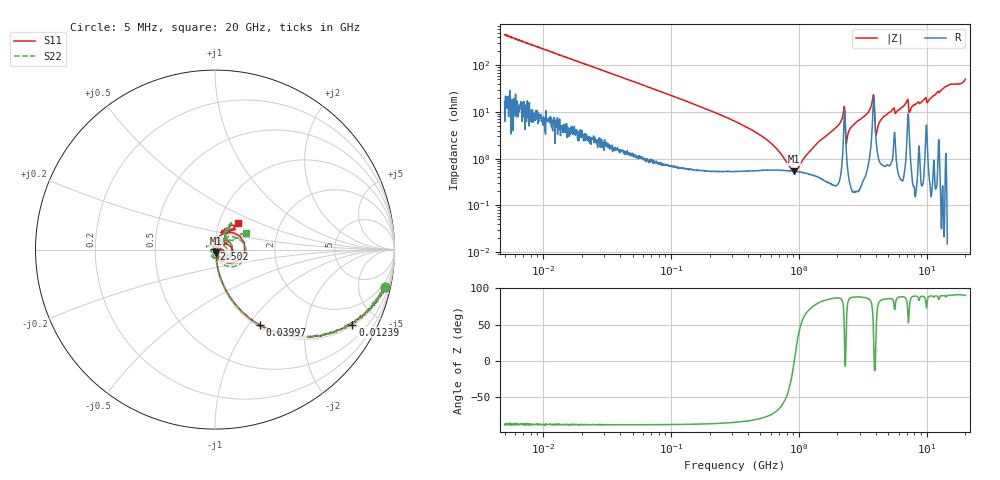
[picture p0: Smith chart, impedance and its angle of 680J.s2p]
!Keysight Technologies,P5008B,MY61100088,A.16.20.02
!Date: Wednesday, November 08, 2023 15:01:09
!Correction: S11(C  2-Port  )
!S21(C  2-Port  )
!S12(C  2-Port  )
!S22(C  2-Port  )
!S2P File: Measurements: S11, S21, S12, S22:Log Frequency Sweep
# Hz S  dB  R 50
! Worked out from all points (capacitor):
!   1601 points, 5 MHz to 20 GHz, reference 50 ohm
!   read as one part in series: C = 71.1 pF near 5.212 MHz
!   lowest |Z| = 536 mohm at 920 MHz (marker M1)
!   series resonance near 919.4 MHz, so ESL is about 420 pH
!   S11 on the Smith chart (normalised r, x): 5 MHz: 1.33, -8.99; 12.39 MHz: 1.04, -3.64; 39.97 MHz: 1.03, -1.14; 2.502 GHz: 0.99, +0.01; 20 GHz: 1.23, +0.38
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5000000  -0.28 -12.4  -13.33 75.4  -13.34 75.4  -0.28 -12.4
1.238641e7  -1.19 -28.7  -6.39 60.7  -6.39 60.7  -1.19 -28.7
1.995555e7  -2.60 -40.8  -3.70 47.8  -3.70 47.8  -2.60 -40.8
3.99702e7  -6.20 -59.4  -1.31 29.2  -1.31 29.2  -6.20 -59.5
7.964482e7  -11.26 -72.7  -0.40 15.7  -0.41 15.7  -11.28 -72.8
3.162278e8  -23.25 -81.5  -0.07 3.3  -0.07 3.3  -23.59 -83.0
9.199521e8  -33.80 -74.9  -0.06 -0.9  -0.06 -0.9  -39.30 -81.7
1.2621e9  -38.61 -74.0  -0.06 -2.1  -0.07 -2.1  -59.34 -157.5
1.669795e9  -62.64 -141.6  -0.07 -3.4  -0.07 -3.4  -40.15 104.6
2.22067e9  -25.05 68.4  -0.27 -7.2  -0.27 -7.2  -24.72 64.0
2.501864e9  -43.45 135.8  -0.08 -4.7  -0.09 -4.7  -47.20 125.2
3.787623e9  -17.03 41.0  -0.96 -13.3  -0.96 -13.3  -17.15 28.1
4.588432e9  -56.45 139.0  -0.06 -9.2  -0.06 -9.2  -35.88 -15.9
5.037181e9  -43.09 95.3  -0.05 -10.7  -0.06 -10.7  -34.05 14.8
5.529816e9  -31.64 29.3  -0.22 -12.6  -0.23 -12.6  -28.34 15.9
6.102182e9  -47.91 -38.1  -0.04 -13.1  -0.04 -13.1  -46.11 24.2
7.165971e9  -19.92 -17.1  -0.77 -14.5  -0.78 -14.5  -23.25 -36.5
8.1999e9  -36.62 -66.6  -0.01 -17.8  -0.02 -17.8  -36.95 -129.9
1.008928e10  -26.34 -68.7  -0.14 -21.0  -0.15 -21.0  -26.81 -96.1
1.096177e10  -39.00 -17.6  0.01 -24.5  0.01 -24.5  -54.49 72.2
1.369891e10  -17.02 52.2  -0.04 -32.0  -0.04 -32.0  -17.35 60.3
2e10  -14.07 49.0  -0.20 -52.8  -0.21 -52.8  -14.17 27.6
